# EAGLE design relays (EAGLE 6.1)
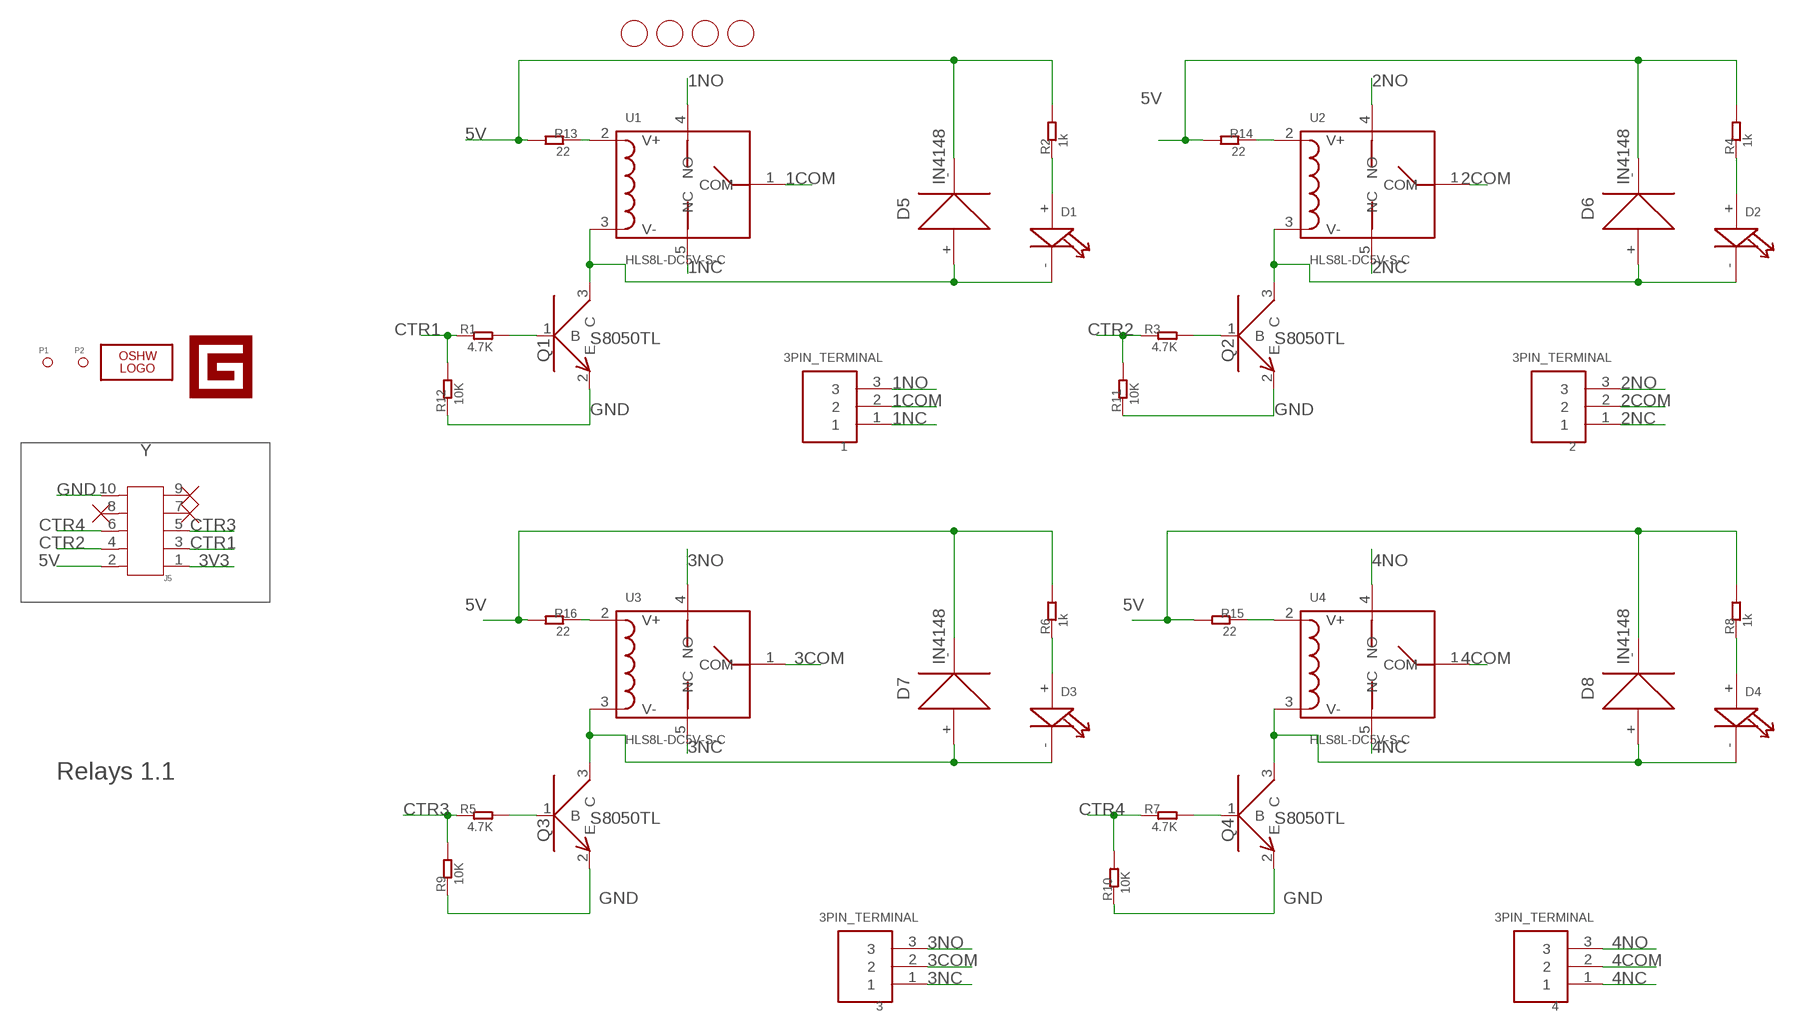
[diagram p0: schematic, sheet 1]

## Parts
1  3PIN_TERMINAL  [3PIN_TERMINAL]
2  3PIN_TERMINAL  [3PIN_TERMINAL]
3  3PIN_TERMINAL  [3PIN_TERMINAL]
4  3PIN_TERMINAL  [3PIN_TERMINAL]
D1  LED0805  [LED0805]
D2  LED0805  [LED0805]
D3  LED0805  [LED0805]
D4  LED0805  [LED0805]
D5  IN4148  DIODE1206  [DIODE1206]
D6  IN4148  DIODE1206  [DIODE1206]
D7  IN4148  DIODE1206  [DIODE1206]
D8  IN4148  DIODE1206  [DIODE1206]
J5  HEADER-SHF-105-01-L-D-SM  [SHF-105-01-L-D-SM]
LOGO1  LOGO-OSHW-FILLX0150-NT  [OSHW_FILLX150_NOTEXT]
P1  PAD-MARK  [ROUND-MARK-0.635]
P2  PAD-MARK  [ROUND-MARK-0.635]
Q1  NPN_9013  [SOT23]
Q2  NPN_9013  [SOT23]
Q3  NPN_9013  [SOT23]
Q4  NPN_9013  [SOT23]
R1  4.7K  R0603  [0603]
R2  1k  R0603  [0603]
R3  4.7K  R0603  [0603]
R4  1k  R0603  [0603]
R5  4.7K  R0603  [0603]
R6  1k  R0603  [0603]
R7  4.7K  R0603  [0603]
R8  1k  R0603  [0603]
R9  10K  R0603  [0603]
R10  10K  R0603  [0603]
R11  10K  R0603  [0603]
R12  10K  R0603  [0603]
R13  22  R0603  [0603]
R14  22  R0603  [0603]
R15  22  R0603  [0603]
R16  22  R0603  [0603]
U1  HLS8L-DC5V-S-C  RELAY  [5P-LEADED-17X21.6]
U2  HLS8L-DC5V-S-C  RELAY  [5P-LEADED-17X21.6]
U3  HLS8L-DC5V-S-C  RELAY  [5P-LEADED-17X21.6]
U4  HLS8L-DC5V-S-C  RELAY  [5P-LEADED-17X21.6]
U$1  PAD-HOLE'3.2/7.0'  [HOLE-D-3.2/7.0]
U$2  PAD-HOLE'3.2/7.0'  [HOLE-D-3.2/7.0]
U$3  PAD-HOLE'3.2/7.0'  [HOLE-D-3.2/7.0]
U$4  PAD-HOLE'3.2/7.0'  [HOLE-D-3.2/7.0]
U$5  LOGO-GADGETEER-NORMAL  [GADGETEER-SILK]

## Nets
1COM: 1.2 U1.1(COM)
1NC: 1.1 U1.5(NC)
1NO: 1.3 U1.4(NO)
2COM: 2.2 U2.1(COM)
2NC: 2.1 U2.5(NC)
2NO: 2.3 U2.4(NO)
3COM: 3.2 U3.1(COM)
3NC: 3.1 U3.5(NC)
3NO: 3.3 U3.4(NO)
3V3: J5.1
4COM: 4.2 U4.1(COM)
4NC: 4.1 U4.5(NC)
4NO: 4.3 U4.4(NO)
5V: D5.- D6.- D7.- D8.- J5.2 R2.2 R4.2 R6.2 R8.2 R13.2 R14.2 R15.2 R16.2
CTR1: J5.3 R1.1 R12.2
CTR2: J5.4 R3.1 R11.2
CTR3: J5.5 R5.1 R9.2
CTR4: J5.6 R7.1 R10.2
GND: J5.10 Q1.2(E) Q2.2(E) Q3.2(E) Q4.2(E) R9.1 R10.1 R11.1 R12.1
N$1: R13.1 U1.2(V+)
N$2: Q1.1(B) R1.2
N$3: D2.+ R4.1
N$4: Q2.1(B) R3.2
N$5: D3.+ R6.1
N$6: D3.- D7.+ Q3.3(C) U3.3(V-)
N$7: D4.+ R8.1
N$8: Q4.1(B) R7.2
N$9: D2.- D6.+ Q2.3(C) U2.3(V-)
N$10: Q3.1(B) R5.2
N$11: R14.1 U2.2(V+)
N$12: D1.- D5.+ Q1.3(C) U1.3(V-)
N$13: D1.+ R2.1
N$14: R15.1 U4.2(V+)
N$15: R16.1 U3.2(V+)
N$18: D4.- D8.+ Q4.3(C) U4.3(V-)
Unconnected: J5.7 J5.8 J5.9

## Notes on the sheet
- S8050TL | S8050TL
- Y
- Relays 1.1
- S8050TL | S8050TL

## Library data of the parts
1-4 = Seeed:3PIN_TERMINAL
D1-D4 = CPT_SMD:LED0805
D5-D8 = CPT_SMD:DIODE
J5 = Connector:HEADER-SHF-105-01-L-D-SM
LOGO1 = Logo:LOGO-OSHW-FILL
P1 P2 = Discreter:PAD-MARK
Q1-Q4 = CPT_SMD:NPN_9013
R1-R16 = CPT_SMD:R0603
U1-U4 = Discreter:RELAY
U$1-U$4 = Discreter:PAD-HOLE
U$5 = Logo:LOGO-GADGETEER

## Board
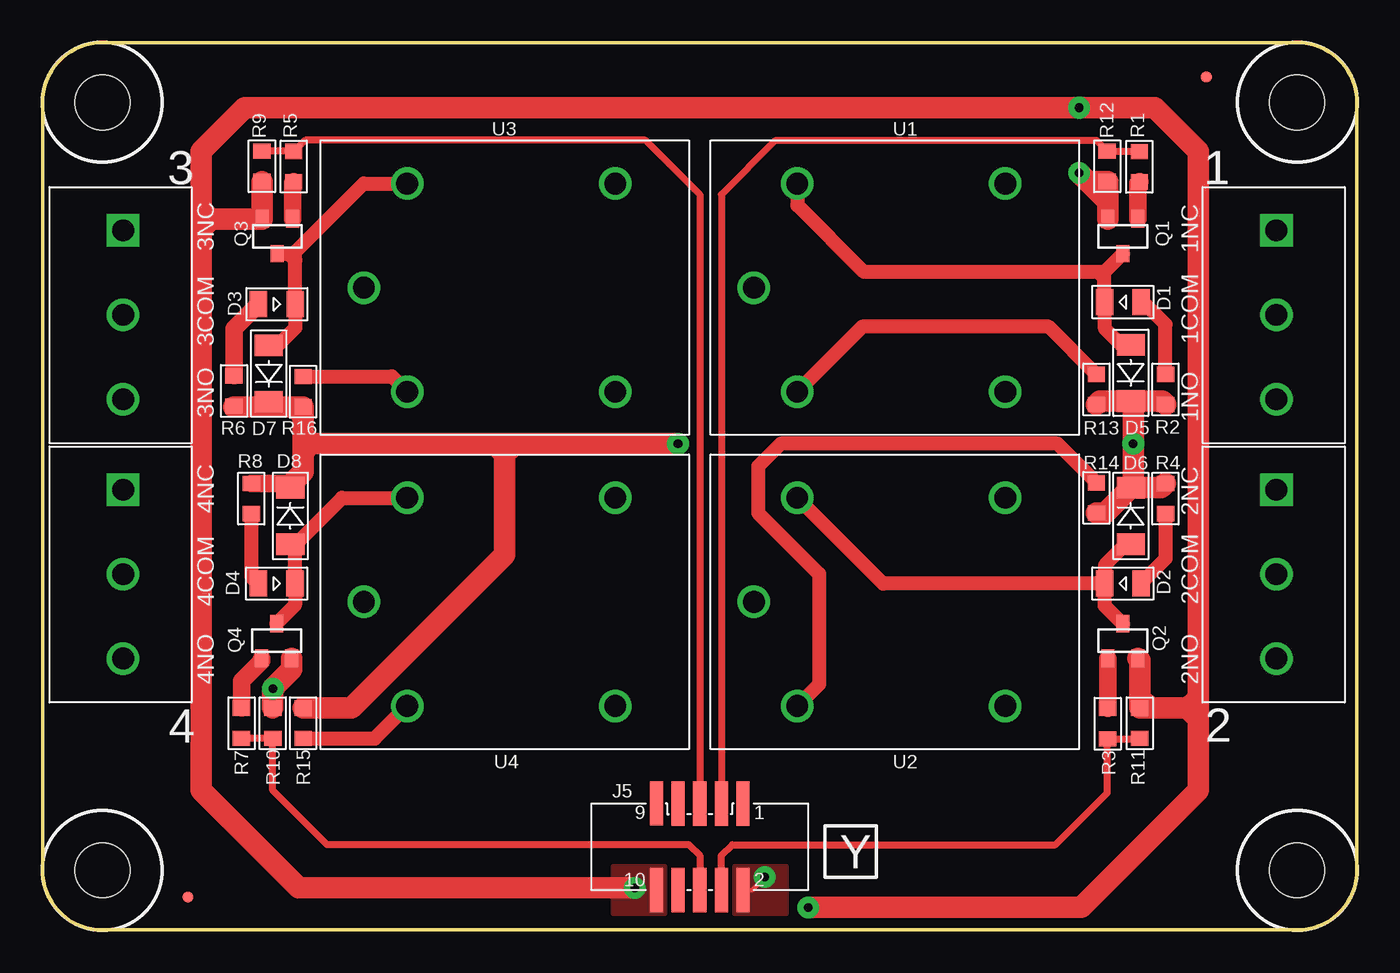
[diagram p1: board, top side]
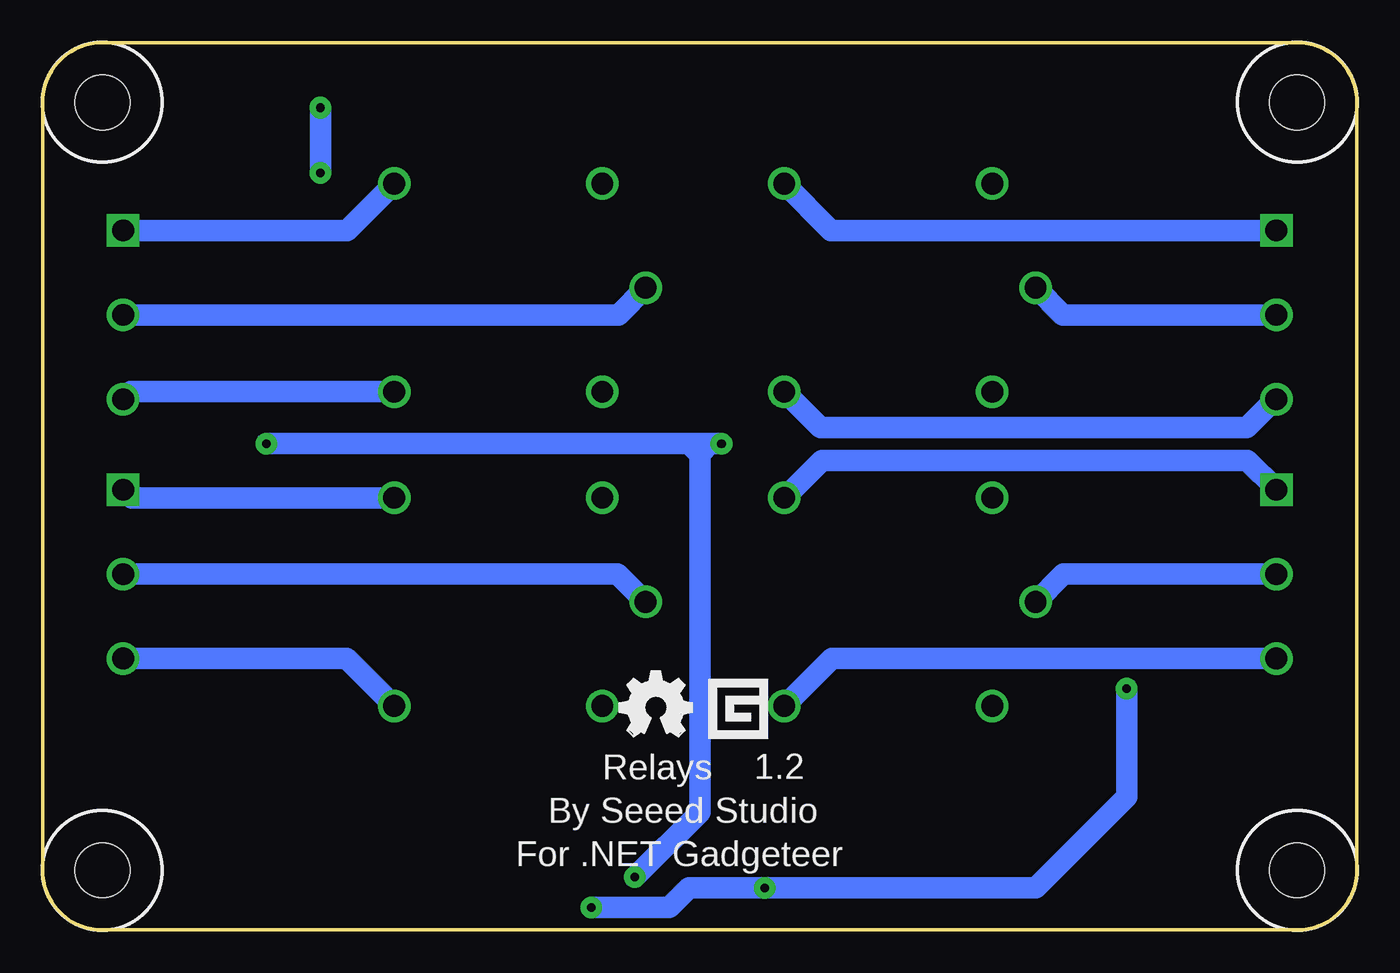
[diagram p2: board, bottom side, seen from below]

Size 77 x 52 mm. Coordinates in mm from the lower left corner, seen from the top.
Outline: 0,48.5 arc-90 3.5,52 73.5,52 arc-90 77,48.5 77,3.5 arc-90 73.5,0 3.5,0 arc-90 0,3.5 0,48.5
Copper layers (1*16): Top 0.035mm / dielectric 1.5mm / Bottom 0.035mm
Design rules: minimum track width 7mil, minimum drill 12mil, track to track 8mil, track to pad 8mil, pad to pad 8mil, via to via 8mil, smd to smd 8mil, copper to edge 20mil, drill to drill 8mil, minimum pad ring 10mil, minimum via ring 8mil, stop-mask expansion 4mil, vias tented up to drill 100mil, thermal gap 10mil

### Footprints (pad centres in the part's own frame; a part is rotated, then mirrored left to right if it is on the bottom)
3PIN_TERMINAL = drill 1.27 pad 1.778 square: 1 0,0 | drill 1.27 pad 1.778: 2 0,4.95; 3 0,9.893
LED0805 = smd 1.016 x 1.524: + -1.077,0; - 1.077,0
DIODE1206 = smd 1.27 x 1.651: + -1.651,0; - 1.651,0
SHF-105-01-L-D-SM = smd 0.762 x 2.6: 1 -2.54,-2.54; 2 -2.54,2.54; 3 -1.27,-2.54; 4 -1.27,2.54; 5 0,-2.54; 6 0,2.54; 7 1.27,-2.54; 8 1.27,2.54; 9 2.54,-2.546; 10 2.54,2.54
ROUND-MARK-0.635 = smd 0.635 x 0.635: P$1 0,0
SOT23 = smd 0.762 x 1.016: 1 -0.889,-1.016; 2 0.889,-1.016; 3 0,1.016
0603 = smd 0.889 x 1.016: 1 -0.889,0; 2 0.889,0
5P-LEADED-17X21.6 = drill 1.27: 1 -2.54,-6.096; 2 0,-12.192; 3 0,0; 4 12.192,-12.192; 5 12.192,0
HOLE-D-3.2/7.0 = hole 3.2: 0,0

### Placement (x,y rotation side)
1  72.28,41 180 top
2  72.28,25.81 180 top
3  4.72,41 180 top
4  4.72,25.81 180 top
D1  63.29,36.8 180 top
D2  63.29,20.3 180 top
D3  13.72,36.67 0 top
D4  13.71,20.3 0 top
D5  63.76,32.65 270 top
D6  63.76,24.27 90 top
D7  13.24,32.61 270 top
D8  14.51,24.27 90 top
J5  38.5,4.88 180 top
LOGO1  43.2,11.36 0 bottom
P1  8.51,1.94 0 top
P2  68.18,50 0 top
Q1  63.29,40.65 180 top
Q2  63.29,16.94 0 top
Q3  13.75,40.65 180 top
Q4  13.71,16.94 0 top
R1  64.26,44.73 270 top
R2  65.79,31.68 270 top
R3  62.4,12.09 90 top
R4  65.79,25.28 90 top
R5  14.71,44.74 270 top
R6  11.21,31.59 270 top
R7  11.65,12.12 90 top
R8  12.23,25.28 90 top
R9  12.85,44.76 90 top
R10  13.48,12.12 270 top
R11  64.28,12.12 270 top
R12  62.38,44.76 90 top
R13  61.74,31.68 270 top
R14  61.74,25.32 270 top
R15  15.26,12.12 90 top
R16  15.26,31.55 270 top
U1  44.22,43.74 0 top
U2  44.22,25.32 0 top
U3  21.36,43.74 0 top
U4  21.36,25.32 0 top
U$1  73.5,48.5 0 top
U$2  73.5,3.5 0 top
U$3  3.5,48.5 0 top
U$4  3.5,3.5 0 top
U$5  35.83,13.39 0 bottom

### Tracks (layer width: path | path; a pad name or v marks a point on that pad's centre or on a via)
1COM
  Bottom 1.27: 1.2 43.27,36.05 U1.1
1NC
  Bottom 1.27: 1.1 59.15,41 U1.5
1NO
  Bottom 1.27: U1.4 71.84,31.55 1.3
2COM
  Bottom 1.27: 2.2 43.3,20.86 U2.1
2NC
  Bottom 1.27: U2.5 71.77,25.32 72.26,25.81 2.1
2NO
  Bottom 1.27: 2.3 59.19,15.91 U2.4
3COM
  Bottom 1.27: 3.2 17.22,36.05 U3.1
3NC
  Bottom 1.27: 3.1 30.8,41 U3.5
3NO
  Bottom 1.27: 3.3 4.78,31.1 6.44,29.44 31.44,29.44 U3.4
4COM
  Bottom 1.27: 4.2 17.19,20.86 U4.1
4NC
  Bottom 1.27: 4.1 4.72,25.83 6.41,27.52 31.35,27.52 U4.5
4NO
  Bottom 1.27: 4.3 30.77,15.91 U4.4
5V  (via drill 0.51 pad 1.27)
  Top 0.254: J5.2 41.55,2.34 v42.31,3.1
  Top 0.813: R6.2 11.66,30.7 11.7,30.66 12.95,30.66 D7.- | 65.81,30.79 R2.2
  Top 1.016: R8.2 14.26,26.17 D8.-
  Top 1.27: 11.2,30.66 11.7,30.66 R16.2 15.26,30.15 | R15.2 18.09,13.01 27.07,21.99 27.07,27.86 | 27.07,27.86 27.07,28.5 | 15.26,30.15 15.26,28.5 | 15.26,28.5 15.26,27.99 | 15.26,27.99 15.26,26.85 14.37,25.96 14.47,25.96 D8.- | 27.07,28.5 26.44,28.5 | 26.44,28.5 15.77,28.5 | 15.77,28.5 15.26,28.5 | 27.07,28.5 v37.23,28.5 | D6.- 63.9,26.06 v63.9,28.5 63.9,30.86 D5.- | D6.- 65.54,25.92 R4.2 | R14.2 62.28,24.44 D6.- | D5.- 61.95,31 R13.2 | D5.- 65.59,31 65.81,30.79 | 27.07,27.86 26.44,28.5 | 27.07,27.86 27.58,28.37 | 15.77,28.5 15.39,28.88 | 15.77,28.5 15.26,27.99 | 15.26,30.15 14.88,30.53
  Bottom 1.27: v42.31,3.1 38.5,6.91 38.5,27.23 38.5,27.86 | 38.5,27.86 38.5,28.5 | v37.23,28.5 37.87,28.5 | 37.87,28.5 38.5,28.5 | 38.5,28.5 39.13,28.5 | 39.13,28.5 v63.9,28.5 | 38.5,27.86 37.87,28.5 | 38.5,27.86 39.13,28.5
  pour Top (no thermals): 40.53,3.73 43.58,3.73 43.58,0.94 40.53,0.94
CTR1
  Top 0.406: J5.3 39.77,43.11 42.95,46.28 61.74,46.28 R12.2 64.23,45.64 R1.1
CTR2
  Top 0.406: J5.4 39.77,4.37 40.41,5 59.35,5 62.38,8.03 62.38,11.18 R3.1 64.26,11.2 R11.2
CTR3
  Top 0.406: J5.5 38.5,43.11 35.33,46.28 15.39,46.28 14.74,45.63 R5.1 12.86,45.63 R9.2
CTR4
  Top 0.406: J5.6 38.5,4.37 37.87,5 16.66,5 13.48,8.18 R10.2 R7.1
GND  (via drill 0.51 pad 1.27)
  Top 1.27: R9.1 12.86,43.85 Q3.2 9.88,41.67 | Q4.2 14.6,15.27 v13.48,14.15 R10.1 | 64.28,13.64 R11.1 64.92,13.01 | 64.28,13.64 64.28,15.82 Q2.2 | v34.69,2.46 15,2.46 9.29,8.18 9.29,41.84 | 9.29,41.84 9.29,42.22 | 9.29,42.22 9.29,45.64 11.83,48.19 v60.73,48.19 65.17,48.19 67.71,45.64 67.71,13.26 | 67.71,13.26 67.71,8.18 60.85,1.32 v44.85,1.32 | 9.84,41.67 9.46,41.67 9.29,41.84 | 67.08,13.01 67.46,13.01 67.71,13.26 | Q1.2 62.4,43.84 R12.1 61.23,43.87 | 61.23,43.87 v60.73,44.38 | 61.23,43.87 62.38,42.72 | 67.08,13.01 67.58,13.51 | 64.92,13.01 67.08,13.01 | 67.08,13.01 67.58,12.5 | 64.92,13.01 64.28,13.64 | 9.88,41.67 9.84,41.67 | 9.84,41.67 9.29,42.22 | 9.88,41.67 9.42,41.2
  Bottom 1.27: v13.48,14.15 13.48,7.8 18.82,2.46 v34.69,2.46 39.13,2.46 40.28,1.32 v44.85,1.32 | v60.73,44.38 v60.73,48.19
  pour Top (isolate 0.254, no thermals): 33.42,3.73 36.47,3.73 36.47,0.94 33.42,0.94
  pour Bottom: -6.59,53.27 -5.31,53.27 -5.31,50.73 -6.59,50.73
N$1
  Top 0.813: R13.1 58.95,35.36 48.02,35.36 U1.2
N$2
  Top 1.016: Q1.1 64.18,43.77 R1.2 64.28,43.87
N$3
  Top 0.813: R4.1 65.79,21.75 64.28,20.24 64.41,20.24 64.41,20.26 D2.+
N$4
  Top 1.016: Q2.1 R3.2
N$5
  Top 1.016: R6.1 11.21,35.24 D3.+
N$6
  Top 0.813: D7.+ 13.78,34.26 14.8,35.28 D3.- 14.8,39.25 | 14.8,39.25 14.8,39.72 | Q3.3 14.71,39.63 14.8,39.72 | 14.8,39.72 18.82,43.74 U3.3 | 14.8,39.25 14.5,39.55
N$7
  Top 0.813: R8.1 12.23,20.7 D4.+
N$8
  Top 1.016: R7.2 11.65,14.61 12.82,15.78 Q4.1
N$9
  Top 0.813: D2.- 62.21,19.01 63.27,17.96 Q2.3 | D6.+ 63.48,22.62 62.25,21.39 62.25,20.33 D2.- | D2.- 49.24,20.3 U2.3
N$10
  Top 1.016: Q3.1 14.64,43.78 R5.2
N$11
  Top 0.813: R14.1 59.45,28.5 43.25,28.5 41.92,27.17 41.92,24.44 45.48,20.88 45.48,14.4 U2.2
N$12
  Top 0.61: 62.21,38.56 61.64,38.56 61.61,38.53 61.74,38.53 62.25,38.02
  Top 0.813: D5.+ 63.18,34.3 62.25,35.23 62.25,36.76 D1.- 62.21,38.56 | 62.21,38.56 Q1.3 | 62.21,38.56 48.13,38.56 44.22,42.47 U1.3
N$13
  Top 0.813: R2.1 65.79,35.5 64.49,36.8 D1.+
N$14
  Top 0.813: R15.1 19.45,11.23 U4.2
N$15
  Top 0.813: R16.1 20.47,32.44 U3.2
N$18
  Top 0.813: Q4.3 14.79,19.04 D4.- 14.79,22.34 | 14.79,22.34 D8.+ | 14.79,22.34 14.79,22.57 17.55,25.32 U4.3

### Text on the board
tPlace: 3NC | 1NC | 3COM | 1COM | 3NO | 1NO | 4NC | 2NC | 2COM | 4COM | 4NO | 2NO | Y
bPlace: 1.2 | Relays | By Seeed Studio | For .NET Gadgeteer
